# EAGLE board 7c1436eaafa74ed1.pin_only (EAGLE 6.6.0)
REV: B

Size 25.4 x 29.21 mm. Coordinates in mm from the lower left corner, seen from the top.
Outline: 25.4,29.21 25.4,2.54 arc-90 22.86,0 2.54,0 arc-90 0,2.54 0,26.67 arc-90 2.54,29.21 25.4,29.21
Copper layers (1*16): Top 0.035mm / dielectric 1.5mm / Bottom 0.035mm
Design rules "adafruit *": minimum track width 8mil, minimum drill 15.5mil, track to track 8mil, track to pad 8mil, pad to pad 8mil, via to via 8mil, smd to smd 8mil, copper to edge 10mil, drill to drill 8mil, minimum pad ring 10mil, minimum via ring 8mil, stop-mask expansion 2mil, vias tented up to drill 20mil, thermal gap 10mil

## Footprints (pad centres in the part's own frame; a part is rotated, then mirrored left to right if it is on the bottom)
0805-NO = smd 1.24 x 1.5: 1 -0.95,0; 2 0.95,0
FIDUCIAL_1MM = smd 1 x 1: 1 0,0
1X05_ROUND_70 = drill 1 pad 1.778: 1 -5.08,0; 2 -2.54,0; 3 0,0; 4 2.54,0; 5 5.08,0
1X01_ROUND = drill 1 pad 1.676: 1 0,0
1X09_ROUND_70 = drill 1 pad 1.778: 1 -10.16,0; 2 -7.62,0; 3 -5.08,0; 4 -2.54,0; 5 0,0; 6 2.54,0; 7 5.08,0; 8 7.62,0; 9 10.16,0
RFMHCW_SMT = smd 2 x 0.8: 1P 8.1,-7; 2P 8.1,-5; 3P 8.1,-3; 4P 8.1,-1; 5P 8.1,1; 6P 8.1,3; 7P 8.1,5; 8P 8.1,7; 9P -8.1,7; 10P -8.1,5; 11P -8.1,3; 12P -8.1,1; 13P -8.1,-1; 14P -8.1,-3; 15P -8.1,-5; 16P -8.1,-7
TSSOP16 = smd 0.305 x 0.991: 1 -2.275,-2.918; 2 -1.625,-2.918; 3 -0.975,-2.918; 4 -0.325,-2.918; 5 0.325,-2.918; 6 0.975,-2.918; 7 1.625,-2.918; 8 2.275,-2.918; 9 2.275,2.918; 10 1.625,2.918; 11 0.975,2.918; 12 0.325,2.918; 13 -0.325,2.918; 14 -0.975,2.918; 15 -1.625,2.918; 16 -2.275,2.918
SOT23-5 = smd 0.55 x 1.2: 1 -0.95,-1.3; 2 0,-1.3; 3 0.95,-1.3; 4 0.95,1.3; 5 -0.95,1.3
SMA_EDGELAUNCH_UFL = smd 4.064 x 1.524: GND@1 2.032,-2.54; GND@2 2.032,2.54 | smd 4.064 x 1.524 bottom: GND@3 2.032,2.54; GND@4 2.032,-2.54 | smd 2.032 x 1.016: P 3.048,0

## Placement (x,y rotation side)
C1  10uF  [0805-NO]  1.78,13.21 270 top
C2  0.1uF  [0805-NO]  15.24,26.92 90 top
C3  10uF  [0805-NO]  2.16,5.59 0 top
FID1  FIDUCIAL""  [FIDUCIAL_1MM]  20.95,9.14 90 top
FID2  FIDUCIAL""  [FIDUCIAL_1MM]  7.49,15.75 90 top
JP1  [1X05_ROUND_70]  7.37,27.94 0 top
JP2  [1X01_ROUND]  21.34,24.51 0 top
JP3  [1X09_ROUND_70]  12.45,2.54 0 top
R1  100K  [0805-NO]  5.08,6.6 270 top
R2  100K  [0805-NO]  5.08,10.03 270 top
R3  100K  [0805-NO]  4.45,12.57 180 top
U1  RFM69HCW  [RFMHCW_SMT]  14.48,14.73 90 top
U2  74HC4050D  [TSSOP16]  3.05,18.54 180 top
U3  AP2112K-3.3  [SOT23-5]  2.29,9.02 0 top
U$8  [ADAFRUIT_3.5MM]  1.4,22.23 0 top
U$14  [PCBFEAT-REV-040]  1.78,14.99 0 bottom
U$19  [ADAFRUIT_TEXT_20MM]  20.45,19.05 0 bottom
X1  uFL/SMA  [SMA_EDGELAUNCH_UFL]  21.34,29.08 270 top

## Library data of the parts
C1-C3 JP1-JP3 R1-R3 U1-U3 U$8 U$14 U$19 X1 = microbuilder
FID1 FID2 = microbuilder; BOM: EXCLUDE

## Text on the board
tPlace: G1 | G2 | G3 | G4 | G5 | RFM69HCW Radio | VIN | EN | SCK | MOSI | RST | GND | G0 | MISO | CS
bPlace: GPIO:3V logic | RFM69HCW Radio | +20dBm output | Vin: 3.3-5.5V / SPI logic: 3-5V safe | Node ID# | Freq

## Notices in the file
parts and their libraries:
microbuilder: This work is placed in the public domain, and may be freely used for commercial and non-commercial work with the following conditions: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
